DATA_BLOCK DB 16
TITLE =BLOCK DATA FOR TIMER
AUTHOR : Esposito
FAMILY : EGAL_srl
NAME : DB_TD_OP
VERSION : 0.1


  STRUCT
   Reserve_0 : INT ;
   Reserve_1 : DINT ;
   Reserve_2 : DINT ;
   Reserve_3 : DINT ;
   Reserve_4 : DINT ;
   Reserve_5 : DINT ;
   R_cam_zero_ON : INT ;	//Value start cam zero - write
   R_cam_zero_OFF : INT ;	//Value stop cam zero - write
   R_cam_one_ON : INT ;	//Value start cam one - write
   R_cam_one_OFF : INT ;	//Value stop cam one - write
   R_cam_two_ON : INT ;	//Value start cam two - write
   R_cam_two_OFF : INT ;	//Value stop cam two - write
   R_cam_three_ON : INT ;	//Value start cam three - write
   R_cam_three_OFF : INT ;	//Value stop cam three - write
   Reserve_6 : INT ;
   Reserve_7 : INT ;
   Reserve_8 : INT ;
   Reserve_9 : INT ;
   Reserve_10 : INT ;
   Reserve_11 : INT ;
   R_cam_seven_ON : INT ;	//Value start cam seven - write
   R_cam_seven_OFF : INT ;	//Value stop cam seven - write
   Reserve_12 : INT ;
   Reserve_13 : INT ;
   Reserve_14 : INT ;
   Reserve_15 : INT ;
   Reserve_16 : INT ;
   Reserve_17 : INT ;
   Reserve_18 : INT ;
   Reserve_19 : INT ;
   Reserve_20 : INT ;
   Reserve_21 : INT ;
   Reserve_22 : INT ;
   Reserve_23 : INT ;
   Reserve_24 : INT ;
   Reserve_25 : INT ;
   Reserve_26 : INT ;
   Reserve_27 : INT ;
   Reserve_28 : REAL ;
   Reserve_29 : REAL ;
   Reserve_30 : REAL ;
   Reserve_31 : REAL ;
   Reserve_32 : REAL ;
   Reserve_33 : REAL ;
   Reserve_34 : REAL ;
   Reserve_35 : REAL ;
   Reserve_36 : REAL ;
   Reserve_37 : REAL ;
   Overload_valve_W : REAL ;	//Value set proportional valve, overload adjustment - write
   Reserve_39 : REAL ;
   Balancing_value_W : REAL ;	//Value set air pressure, balancing press - write
   Reserve_41 : REAL ;
   Reserve_42 : REAL ;
   Reserve_43 : REAL ;
   Reserve_44 : REAL ;
   Reserve_45 : REAL ;
   Main_mot_PQW306_W : REAL ;	//Value set main motor in stroke - write
   Reserve_46 : INT ;
   Reserve_47 : INT ;
   Reserve_48 : INT ;
   Reserve_49 : INT ;
   Reserve_50 : INT ;
   Reserve_51 : INT ;
   Reserve_52 : INT ;
   Reserve_53 : INT ;
   Reserve_54 : WORD ;
   Reserve_55 : INT ;
   Reserve_56 : WORD ;
   Reserve_57 : INT ;
   Reserve_58 : WORD ;
   Reserve_59 : INT ;
   Reserve_60 : WORD ;
   Reserve_61 : INT ;
   Num_prog_Rob2_W : INT ;	//Value number program for running, robot 2 - write
   Num_cycle_Rob1_W : INT ;	//Value number cycle for runnig, robot 1  - write
   Num_cycle_Rob2_W : INT ;	//Value number cycle for running, robot 2 - write
   out_PAW304 : REAL ;	//Valore uscita proporz.
   Num_prog_Rob1_W : INT ;	//Value number program for running, robot 1 - write
   Balan_value : INT ;	//Value from OP_37 for Balancing press
   Elec_cam_ON0 : INT ;	//Electrical cam for cycle 00 - ON
   Elec_cam_OFF0 : INT ;	//Electrical cam for cycle 00 - OFF
   Elec_cam_ON1 : INT ;	//Electrical cam for robot 1 start - ON
   Elec_cam_OFF1 : INT ;	//Electrical cam for robot 1 start - OFF
   Elec_cam_ON2 : INT ;	//Electrical cam for robot 2 start - ON
   Elec_cam_OFF2 : INT ;	//Electrical cam for robot 2 start - OFF
   Elec_cam_ON3 : INT ;	//Electrical cam for safety robot 1 - ON
   Elec_cam_OFF3 : INT ;	//Electrical cam for safety robot 1 - OFF
   Elec_cam_ON4 : INT ;	//Electrical cam for safety robot 2 - ON
   Elec_cam_OFF4 : INT ;	//Electrical cam for safety robot 2 - OFF
   Elec_cam_ON5 : INT ;	//Electrical cam spare - ON
   Elec_cam_OFF5 : INT ;	//Electrical cam spare - OFF
   Elec_cam_ON6 : INT ;	//Electrical cam spare - ON
   Elec_cam_OFF6 : INT ;	//Electrical cam spare - OFF
   Main_mot_min : REAL ;	//Minimal speed main motor press
   Main_mot_max : REAL ;	//Maximal speed main motor press
   Mode_press_cycle : INT ;	//Word for visualize the mode of job press
   Elec_cam_ON7 : INT ;	//Spare cam PLC
   Elec_cam_OFF7 : INT ;	//Spare cam PLC
   Elec_cam_ON8 : INT ;	//Spare cam PLC
   Elec_cam_OFF8 : INT ;	//Spare cam PLC
   Elec_cam_ON9 : INT ;	//Spare cam PLC
   Elec_cam_OFF9 : INT ;	//Spare cam PLC
   Elec_cam_ON10 : INT ;	//Spare cam PLC
   Elec_cam_OFF10 : INT ;	//Spare cam PLC
   Elec_cam_ON11 : INT ;	//Spare cam PLC
   Elec_cam_OFF11 : INT ;	//Spare cam PLC
   Elec_cam_ON12 : INT ;	//Spare cam PLC
   Elec_cam_OFF12 : INT ;	//Spare cam PLC
   Elec_Num_prog : INT ;	//Number cam for load data cam PLC
   Elec_Start_prog : INT ;	//Value cam for load data cam PLC
   Elec_Stop_prog : INT ;	//Value cam for load data cam PLC
   K_parts_counter : INT ;	//Value for conters pices press
   Recipe_plc : STRING  [12 ];
  END_STRUCT ;
BEGIN
   Reserve_0 := 0;
   Reserve_1 := L#0;
   Reserve_2 := L#0;
   Reserve_3 := L#0;
   Reserve_4 := L#99999999;
   Reserve_5 := L#99999999;
   R_cam_zero_ON := 0;
   R_cam_zero_OFF := 0;
   R_cam_one_ON := 0;
   R_cam_one_OFF := 0;
   R_cam_two_ON := 0;
   R_cam_two_OFF := 0;
   R_cam_three_ON := 0;
   R_cam_three_OFF := 0;
   Reserve_6 := 0;
   Reserve_7 := 0;
   Reserve_8 := 0;
   Reserve_9 := 0;
   Reserve_10 := 0;
   Reserve_11 := 0;
   R_cam_seven_ON := 0;
   R_cam_seven_OFF := 0;
   Reserve_12 := 0;
   Reserve_13 := 0;
   Reserve_14 := 0;
   Reserve_15 := 0;
   Reserve_16 := 0;
   Reserve_17 := 0;
   Reserve_18 := 0;
   Reserve_19 := 0;
   Reserve_20 := 0;
   Reserve_21 := 100;
   Reserve_22 := 300;
   Reserve_23 := 0;
   Reserve_24 := 0;
   Reserve_25 := 0;
   Reserve_26 := 999;
   Reserve_27 := 15;
   Reserve_28 := 0.000000e+000;
   Reserve_29 := 0.000000e+000;
   Reserve_30 := 0.000000e+000;
   Reserve_31 := 0.000000e+000;
   Reserve_32 := 0.000000e+000;
   Reserve_33 := 0.000000e+000;
   Reserve_34 := 0.000000e+000;
   Reserve_35 := 0.000000e+000;
   Reserve_36 := 0.000000e+000;
   Reserve_37 := 0.000000e+000;
   Overload_valve_W := 0.000000e+000;
   Reserve_39 := 0.000000e+000;
   Balancing_value_W := 0.000000e+000;
   Reserve_41 := 0.000000e+000;
   Reserve_42 := 0.000000e+000;
   Reserve_43 := 0.000000e+000;
   Reserve_44 := 0.000000e+000;
   Reserve_45 := 0.000000e+000;
   Main_mot_PQW306_W := 0.000000e+000;
   Reserve_46 := 0;
   Reserve_47 := 0;
   Reserve_48 := 0;
   Reserve_49 := 0;
   Reserve_50 := 0;
   Reserve_51 := 0;
   Reserve_52 := 0;
   Reserve_53 := 0;
   Reserve_54 := W#16#0;
   Reserve_55 := 0;
   Reserve_56 := W#16#0;
   Reserve_57 := 0;
   Reserve_58 := W#16#0;
   Reserve_59 := 0;
   Reserve_60 := W#16#0;
   Reserve_61 := 0;
   Num_prog_Rob2_W := 1;
   Num_cycle_Rob1_W := 1;
   Num_cycle_Rob2_W := 0;
   out_PAW304 := 0.000000e+000;
   Num_prog_Rob1_W := 0;
   Balan_value := 0;
   Elec_cam_ON0 := 0;
   Elec_cam_OFF0 := 0;
   Elec_cam_ON1 := 0;
   Elec_cam_OFF1 := 0;
   Elec_cam_ON2 := 0;
   Elec_cam_OFF2 := 0;
   Elec_cam_ON3 := 0;
   Elec_cam_OFF3 := 0;
   Elec_cam_ON4 := 0;
   Elec_cam_OFF4 := 0;
   Elec_cam_ON5 := 0;
   Elec_cam_OFF5 := 0;
   Elec_cam_ON6 := 0;
   Elec_cam_OFF6 := 0;
   Main_mot_min := 0.000000e+000;
   Main_mot_max := 0.000000e+000;
   Mode_press_cycle := 0;
   Elec_cam_ON7 := 0;
   Elec_cam_OFF7 := 0;
   Elec_cam_ON8 := 0;
   Elec_cam_OFF8 := 0;
   Elec_cam_ON9 := 0;
   Elec_cam_OFF9 := 0;
   Elec_cam_ON10 := 0;
   Elec_cam_OFF10 := 0;
   Elec_cam_ON11 := 0;
   Elec_cam_OFF11 := 0;
   Elec_cam_ON12 := 0;
   Elec_cam_OFF12 := 0;
   Elec_Num_prog := 0;
   Elec_Start_prog := 0;
   Elec_Stop_prog := 0;
   K_parts_counter := 0;
   Recipe_plc := '';
END_DATA_BLOCK

